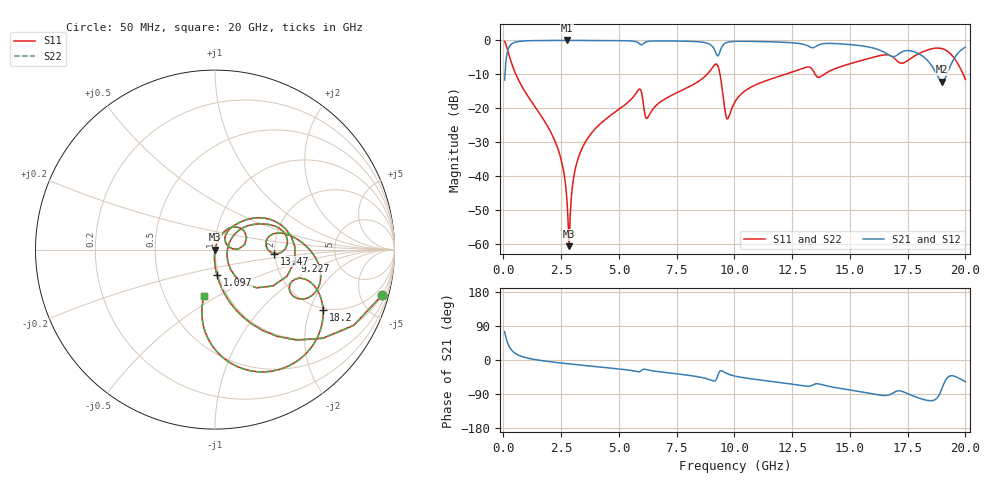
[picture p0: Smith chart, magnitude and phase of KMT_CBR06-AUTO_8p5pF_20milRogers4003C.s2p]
! Data measured by Modelithics Inc. support@modelithics.com 813-866-6335
! KEMET CBR06-AUTO 8.5pF, Pad Width= 0.851mm, Pad Length= 0.64mm, Pad Gap= 0.62mm, 20mil Rogers 4003C substrate Data, January 2022
# hz S ma R 50
! 2 Port Network Data from SP1.SP block
! freq  magS11  angS11  magS21  angS21  magS12  angS12  magS22  angS22
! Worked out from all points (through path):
!   401 points, 50 MHz to 20 GHz, reference 50 ohm
!   highest |S21| = -0.01 dB at 2.743 GHz (marker M1); lowest = -12.2 dB at 19 GHz (marker M2)
!   group delay of S21, straight-line fit = 14.4 ps
!   lowest |S11| = -60.7 dB at 2.843 GHz (marker M3), VSWR 1.00, Z = 50.1 + j0.00693 ohm
!   |S11| at or under -10 dB: 538.5 MHz to 8.815 GHz (8.276 GHz wide, 177 % of centre); 9.376 GHz to 12.2 GHz (2.826 GHz wide, 26.2 % of centre); 13.5 GHz to 13.89 GHz (388.2 MHz wide, 2.84 % of centre)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
!   |S22| runs from -60.7 to -0.3 dB; largest |S21 - S12| = 0
!   S11 on the Smith chart (normalised r, x): 50 MHz: 0.98, -7.35; 1.097 GHz: 0.98, -0.29; 9.227 GHz: 2.55, -0.42; 13.47 GHz: 1.98, -0.10; 18.2 GHz: 1.92, -2.48; 20 GHz: 0.78, -0.44
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5e7  0.9656 -15.2  0.2598 74.7  0.2598 74.7  0.9656 -15.2
3.99125e8  0.4154 -66.8  0.909 23.1  0.909 23.1  0.4154 -66.8
1.097375e9  0.1435 -85.4  0.989 4.3  0.989 4.3  0.1435 -85.4
2.34425e9  0.02599 -95.1  0.9988 -6.9  0.9988 -6.9  0.02599 -95.1
2.74325e9  0.004737 -88.9  0.999 -9.6  0.999 -9.6  0.004737 -88.9
2.843e9  0.0009249 4.3  0.999 -10.2  0.999 -10.2  0.0009249 4.3
3.092375e9  0.01194 73.7  0.9989 -11.8  0.9989 -11.8  0.01194 73.7
3.391625e9  0.02516 74.1  0.9986 -13.6  0.9986 -13.6  0.02516 74.1
5.8355e9  0.1852 40.5  0.9253 -31.0  0.9253 -31.0  0.1852 40.5
6.2345e9  0.07193 35.8  0.9636 -25.9  0.9636 -25.9  0.07193 35.8
6.73325e9  0.1194 55.4  0.9848 -30.9  0.9848 -30.9  0.1194 55.4
8.828e9  0.3196 33.5  0.9107 -49.8  0.9107 -49.8  0.3196 33.5
9.227e9  0.4487 -8.4  0.6189 -50.1  0.6189 -50.1  0.4487 -8.4
9.675875e9  0.06958 -13.0  0.9352 -35.8  0.9352 -35.8  0.06958 -13.0
1.0025e10  0.1247 36.5  0.9682 -42.5  0.9682 -42.5  0.1247 36.5
1.336662e10  0.3762 -1.8  0.7802 -66.7  0.7802 -66.7  0.3762 -1.8
1.346638e10  0.3297 -3.8  0.7924 -63.7  0.7924 -63.7  0.3297 -3.8
1.506238e10  0.4593 7.5  0.8652 -79.7  0.8652 -79.7  0.4593 7.5
1.670825e10  0.6052 -23.7  0.6026 -92.0  0.6026 -92.0  0.6052 -23.7
1.82045e10  0.6906 -29.3  0.5671 -104.5  0.5671 -104.5  0.6906 -29.3
1.90025e10  0.7554 -62.7  0.2468 -72.6  0.2468 -72.6  0.7554 -62.7
2e10  0.2663 -103.1  0.7953 -57.3  0.7953 -57.3  0.2663 -103.1
